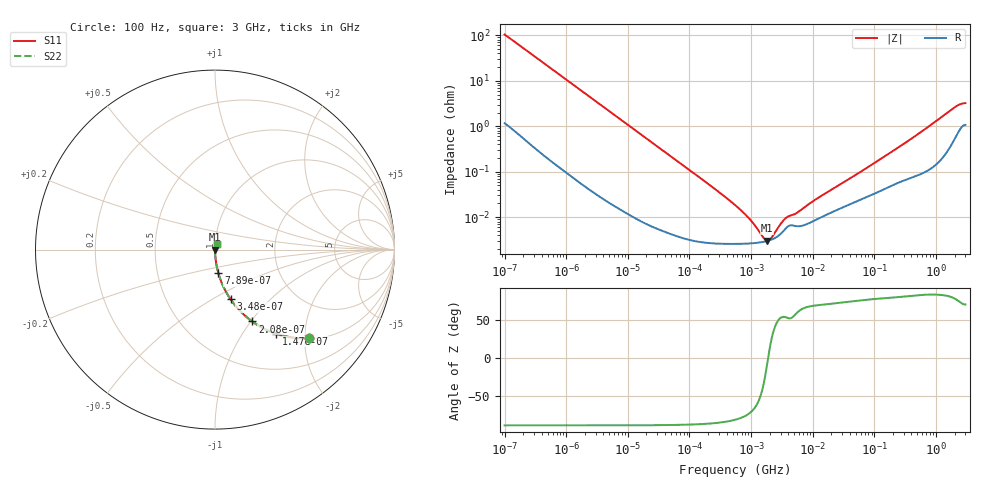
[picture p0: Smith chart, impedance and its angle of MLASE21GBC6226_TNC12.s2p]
! MLASE21GBC6226_TNC12  S-PARAMETER MODEL  ( Standard Model )
! Model Generated by TAIYO YUDEN Corporation (http://www.ty-top.com)
! Version 1.0
! TAIYO YUDEN Control No. 220601
! Copyright(c) 2017 TAIYO YUDEN CO.,LTD. All Rights Reserved.
! Product Description (link to TY-COMPAS)
! https://ds.yuden.co.jp/TYCOMPAS/or/detail?pn=MLASE21GBC6226MTNC12&u=M
! Products Name : Multilayer Ceramic Capacitors
! Characteristics :
!  Capacitance : 22 [uF] , Rated Voltage : 16 [V] , TCC : X6S
!  Case Size : 2.0 x 1.25 / 0.079 x 0.049 [mm/inch] , Thickness : 1.25 / 0.049 [mm/inch]
!  (Conditions: Temperature = 25 [degC] , DC Bias Voltage = 0 [V])
! External Node Assignments :
!  1  o---| |---o  2
! GND o---------o GND
! Frequency Range : 100Hz  -  3GHz  [ 401 STEP ]
# MHZ S RI R 50
! Freq[MHz].  S11 Real  S11 Imag  S21 Real  S21 Imag  S12 Real  S12 Imag  S22 Real  S22 Imag
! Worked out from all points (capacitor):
!   401 points, 100 Hz to 3 GHz, reference 50 ohm
!   read as one part in series: C = 15.1 uF near 109 Hz
!   lowest |Z| = 3.01 mohm at 1.828 MHz (marker M1)
!   series resonance near 1.891 MHz, so ESL is about 470 pH
!   S11 on the Smith chart (normalised r, x): 100 Hz: 1.02, -2.10; 147 Hz: 1.02, -1.43; 208 Hz: 1.01, -1.02; 348 Hz: 1.01, -0.61; 789 Hz: 1.00, -0.27; 3 GHz: 1.02, +0.06
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0.0001  0.5237 -0.4939  0.4763 0.4939  0.4763 0.4939  0.5237 -0.4939
0.000147  0.3397 -0.4682  0.6603 0.4682  0.6603 0.4682  0.3397 -0.4682
0.000208  0.2074 -0.4004  0.7926 0.4004  0.7926 0.4004  0.2074 -0.4004
0.000348  0.0867 -0.2767  0.9133 0.2767  0.9133 0.2767  0.0867 -0.2767
0.000789  0.019 -0.132  0.981 0.132  0.981 0.132  0.019 -0.132
0.001788  0.00408 -0.0595  0.9959 0.0595  0.9959 0.0595  0.00408 -0.0595
0.005476  0.000574 -0.0196  0.9994 0.0196  0.9994 0.0196  0.000574 -0.0196
0.031977  6.47e-05 -0.00339  0.9999 0.00339  0.9999 0.00339  6.47e-05 -0.00339
0.221826  2.69e-05 -0.000487  1 0.000487  1 0.000487  2.69e-05 -0.000487
0.547723  2.57e-05 -0.000183  1 0.000183  1 0.000183  2.57e-05 -0.000183
0.806856  2.6e-05 -0.000111  1 0.000111  1 0.000111  2.6e-05 -0.000111
0.918067  2.63e-05 -9.14e-05  1 9.14e-05  1 9.14e-05  2.63e-05 -9.14e-05
1.827928  2.98e-05 -3.93e-06  1 3.93e-06  1 3.93e-06  2.98e-05 -3.93e-06
3.486191  5.25e-05 7.28e-05  0.9999 -7.28e-05  0.9999 -7.28e-05  5.25e-05 7.28e-05
4.141163  6.48e-05 8.36e-05  0.9999 -8.36e-05  0.9999 -8.36e-05  6.48e-05 8.36e-05
5.597215  6.29e-05 0.000108  0.9999 -0.000108  0.9999 -0.000108  6.29e-05 0.000108
9.794414  7.93e-05 0.000203  0.9999 -0.000203  0.9999 -0.000203  7.93e-05 0.000203
175.1444  0.000474 0.0025  0.9995 -0.0025  0.9995 -0.0025  0.000474 0.0025
513.708  0.00088 0.0067  0.9991 -0.0067  0.9991 -0.0067  0.00088 0.0067
2036.508  0.00606 0.0256  0.9939 -0.0256  0.9939 -0.0256  0.00606 0.0256
2525.516  0.00982 0.0291  0.9902 -0.0291  0.9902 -0.0291  0.00982 0.0291
3000  0.0115 0.0298  0.9885 -0.0298  0.9885 -0.0298  0.0115 0.0298
